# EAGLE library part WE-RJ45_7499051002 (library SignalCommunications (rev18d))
Order Code 7499051002 Design THT xBase-T 10/100 Base-T Ports 1x2 STACKED Application Standard Tab Position UP & DOWN LED (Left-Right) NONE EMI Fingers Yes Details see: http://katalog.we-online.de/en/pbs/WE-LAN_RJ45/7499051002? Updated by Yingchun Shan 2016-08-29 2016(C) Würth Elektronik
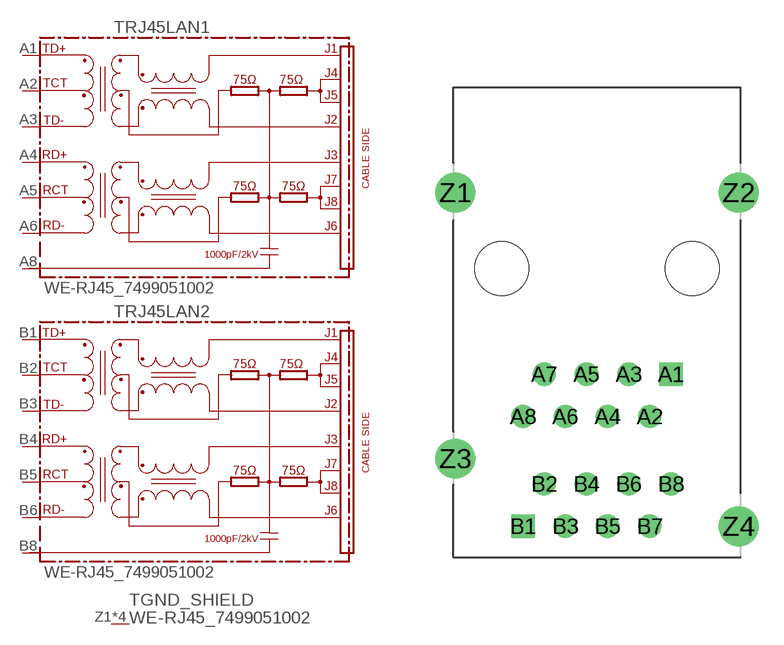
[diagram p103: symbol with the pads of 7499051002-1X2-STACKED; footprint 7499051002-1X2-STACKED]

Designator prefix T; gates RJ45LAN1=74990X-THT-10/100-T RJ45LAN2=74990X-THT-10/100-T GND_SHIELD=GND_PIN

## WE-RJ45_7499051002 (COMPANY-URL: http://www.we-online.de; CREATED-BY: Christin Zierenner; CREATED-DATE: AUG 2012; DATASHEET-URL: http://katalog.we-online.de/kataloge/eisos/media/pdf/7499051002.pdf; MANUFACTURER: Würth Elektronik eiSos GmbH)  [7499051002-1X2-STACKED]
A1  RJ45LAN1:TD+
A2  RJ45LAN1:TCT
A3  RJ45LAN1:TD-
A4  RJ45LAN1:RD+
A5  RJ45LAN1:RCT
A6  RJ45LAN1:RD-
A8  RJ45LAN1:8
B1  RJ45LAN2:TD+
B2  RJ45LAN2:TCT
B3  RJ45LAN2:TD-
B4  RJ45LAN2:RD+
B5  RJ45LAN2:RCT
B6  RJ45LAN2:RD-
B8  RJ45LAN2:8
Z1  GND_SHIELD:1  pwr
Z2  GND_SHIELD:1  pwr
Z3  GND_SHIELD:1  pwr
Z4  GND_SHIELD:1  pwr

## Footprint 7499051002-1X2-STACKED (pad centres in mm)
MAX HEIGHT=25.20mm PORTS----1X2 STACKED LED --No
drill 0.89 square: A1 4.445,-6.35; B1 -4.445,-15.49
drill 0.89: A2 3.175,-8.89; A3 1.905,-6.35; A4 0.635,-8.89; A5 -0.635,-6.35; A6 -1.905,-8.89; A7 -3.175,-6.35; A8 -4.445,-8.89; B2 -3.175,-12.95; B3 -1.905,-15.49; B4 -0.635,-12.95; B5 0.635,-15.49; B6 1.905,-12.95; B7 3.175,-15.49; B8 4.445,-12.95
drill 1.6: Z1 -8.51,4.57; Z2 8.51,4.57; Z3 -8.51,-11.43; Z4 8.51,-15.5
hole 3.25 at 5.715,0
hole 3.25 at -5.715,0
